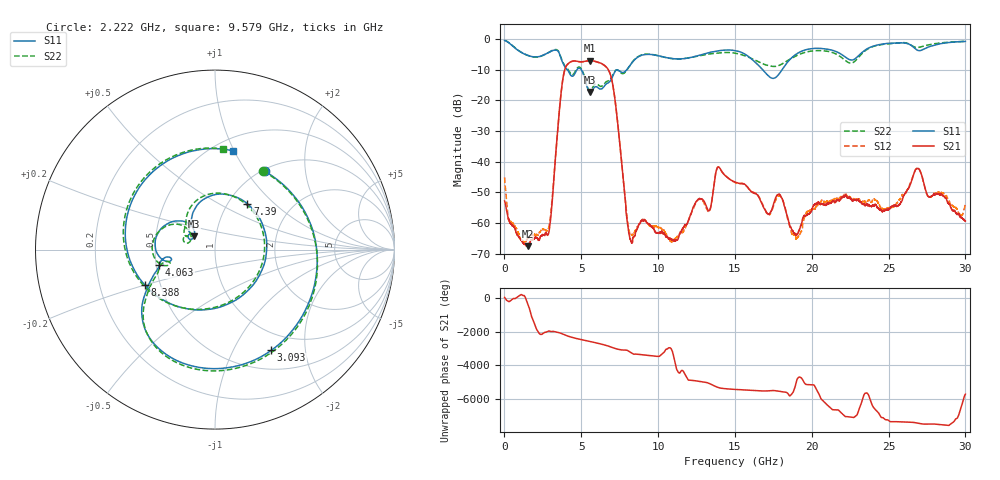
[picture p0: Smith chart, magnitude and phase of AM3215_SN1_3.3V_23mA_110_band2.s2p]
!Agilent Technologies,E8364B,MY43040894,A.07.50.67
!Agilent E8364B: A.07.50.67
!Date: Tuesday, May 25, 2021 15:26:50
!Correction: S11(Full 2 Port(1,2))
!S21(Full 2 Port(1,2))
!S12(Full 2 Port(1,2))
!S22(Full 2 Port(1,2))
!S2P File: Measurements: S11, S21, S12, S22:
# Hz S  dB  R 50
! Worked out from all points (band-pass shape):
!   6401 points, 10 MHz to 30 GHz, reference 50 ohm
!   highest |S21| = -7.02 dB at 5.572 GHz (marker M1); lowest = -67.6 dB at 1.5 GHz (marker M2)
!   |S21| within 3 dB of the highest: 3.923 GHz to 6.766 GHz (2.843 GHz wide, 53.2 % of centre)
!   lowest |S11| = -17.2 dB at 5.558 GHz (marker M3), VSWR 1.32, Z = 39.2 + j5.87 ohm
!   |S11| at or under -10 dB: 4.096 GHz to 4.717 GHz (621.5 MHz wide, 14.1 % of centre); 5.002 GHz to 7.964 GHz (2.962 GHz wide, 45.7 % of centre); 16.81 GHz to 18.07 GHz (1.258 GHz wide, 7.22 % of centre)
!   |S22| runs from -16.8 to -0.5 dB; largest |S21 - S12| = 0.0064
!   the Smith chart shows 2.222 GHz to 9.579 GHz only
!   S11 on the Smith chart (normalised r, x): 2.222 GHz: 1.03, +1.23; 3.093 GHz: 0.75, -1.43; 4.063 GHz: 0.52, -0.10; 7.39 GHz: 1.22, +0.69; 8.388 GHz: 0.41, -0.20; 9.579 GHz: 0.62, +0.99
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1e7  -0.44 -13.5  -52.80 44.7  -45.12 61.5  -0.46 -13.7
5.113953e8  -2.17 -92.9  -60.65 -68.9  -60.27 -15.8  -2.10 -92.8
1.500128e9  -5.27 144.2  -67.55 29.8  -65.30 69.4  -5.29 144.7
2.221762e9  -5.73 57.5  -65.61 104.9  -63.54 82.7  -5.80 58.3
3.093347e9  -3.84 -60.8  -53.87 156.6  -52.82 -147.4  -3.72 -59.3
4.063336e9  -9.83 -164.2  -8.45 -87.3  -8.48 -87.5  -9.47 -159.5
5.009895e9  -10.06 155.5  -7.40 41.6  -7.48 41.5  -9.75 161.1
5.55815e9  -17.24 147.7  -7.03 -66.9  -7.08 -66.9  -16.76 158.0
5.572208e9  -17.23 148.7  -7.02 -69.8  -7.08 -69.8  -16.76 159.0
7.390352e9  -10.10 54.8  -28.32 -174.4  -28.33 -174.0  -10.21 59.6
8.388456e9  -7.17 -153.2  -64.61 -96.1  -63.73 78.2  -7.05 -152.9
9.578684e9  -5.05 79.5  -61.20 154.2  -61.01 67.9  -4.99 85.6
1.000979e10  -5.43 41.7  -63.12 122.8  -61.55 -111.1  -5.43 47.9
1.148586e10  -6.46 -83.7  -62.79 -44.7  -63.18 60.9  -6.43 -78.5
1.29385e10  -4.90 171.4  -52.55 31.0  -52.94 35.1  -5.17 178.8
1.5005e10  -3.74 48.7  -46.63 -52.7  -46.79 -51.8  -4.59 51.8
1.677628e10  -9.82 -61.9  -53.86 -145.2  -53.67 -146.9  -7.98 -80.3
1.810709e10  -9.72 128.6  -52.46 163.4  -52.60 164.4  -7.99 153.6
2.00049e10  -3.10 20.6  -55.52 -138.4  -55.50 -121.3  -3.89 37.8
2.500479e10  -1.37 -57.6  -55.61 -116.8  -55.09 124.0  -1.50 -57.3
2.688854e10  -3.66 -89.1  -42.18 94.4  -42.04 91.3  -2.74 -87.1
3e10  -0.77 -111.7  -59.38 23.8  -53.79 148.3  -0.71 -115.8
